[IBIS Ver]   3.2
[File name]   xc7455a-d.ibs
[File Rev]   0.1
[Date]   Wed Sep 18 11:10:01 CDT 2002
[Source]   File originated at Somerset. Created by Joshua Siegel.
[Notes]   This IBIS model is for the Apollo 483BGA ceramic package.
|   The driver and receiver models are characterized up to
|   2.5V mode on the data bus and 2.5V mode on the L3
|   interface. The convention is apollox.ibs, where x
|   is one of the configurations of data bus/L3 bus voltage
|   modes. Following is a table of the code for bus combinations:
|   IBIS model   Bus mode   L3 mode
|   xc7455a-a.ibs  2.5V   2.5V
|   xc7455a-b.ibs  2.5V   1.8V
|   xc7455a-c.ibs  2.5V   1.5V
|   xc7455a-d.ibs  1.8V   2.5V
|   xc7455a-e.ibs  1.8V   1.8V
|   xc7455a-f.ibs  1.8V   1.5V
|   NOTE: Pullup and pulldown data are non-monotonic.
|   It is safe to ignore non-monotonicity warnings.
[Disclaimer]   This information is for modeling purposes only and
|   is not guaranteed.
[Component]   Apollo
[Manufacturer]  Motorola
[Package]
|   typ   min   max
R_pkg   0.990   0.111   1.910
L_pkg   6.110nH   0.540nH   12.0nH
C_pkg   2.170pF   0.370pF   4.36pF
[Pin]   signal_name   model_name  R_pin   L_pin   C_pin
A02   PLL_CFG0   busio   1.775   1.11e-08   3.54e-12
A03   HRESET_   busio   1.555   9.71e-09   3.04e-12
A04   L3VSEL   rcvr   1.545   9.6e-09   3.9e-12
A05   TT3   busio   1.355   8.48e-09   2.8e-12
A06   A8   busio   1.436   8.97e-09   2.82e-12
A07   A6   busio   1.404   8.71e-09   3.56e-12
A09   DX_   busio   1.099   6.81e-09   2.27e-12
A10   A10   busio   1.065   6.59e-09   2.2e-12
A12   L3_DATAP7   l3io   1.065   6.56e-09   2.72e-12
A13   L3_DATA61   l3io   1.046   6.47e-09   2.17e-12
A14   L3_DATA57   l3io   1.117   6.96e-09   2.86e-12
A15   L3_DATAP6   l3io   1.113   6.9e-09   2.3e-12
A16   L3_DATA53   l3io   1.277   7.98e-09   3.25e-12
A17   L3_DATA52   l3io   1.227   7.62e-09   2.51e-12
A18   L3_DATA48   l3io   1.428   8.89e-09   3.6e-12
A19   L3_DATA47   l3io   1.447   9.04e-09   2.84e-12
A20   L3_DATA44   l3io   1.484   9.26e-09   2.99e-12
A21   L3_DATA41   l3io   1.541   9.62e-09   3.1e-12
A22   GND   POWER   0   0   0
B01   GND   POWER   0   0   0
B02   AVDD   POWER   1.462   9.13e-09   2.87e-12
B03   OVDD   POWER   0   0   0
B04   PMON_OUT_   busio   1.396   8.7e-09   2.83e-12
B05   GND   POWER   0   0   0
B06   OSHD_   busio   1.394   8.56e-09   3.06e-12
B07   TBST_   busio   1.91   1.198e-08   4.06e-12
B08   MCP_   busio   1.139   7.1e-09   2.91e-12
B09   EXT_QUAL   busio   0.962   5.94e-09   2.01e-12
B10   CHKS_   busio   0.928   5.73e-09   1.95e-12
B12   GND   POWER   0   0   0
B13   GVDD   POWER   0   0   0
B14   GND   POWER   0   0   0
B15   GVDD   POWER   0   0   0
B16   GND   POWER   0   0   0
B17   GVDD   POWER   0   0   0
B18   GND   POWER   0   0   0
B19   GVDD   POWER   0   0   0
B20   GND   POWER   0   0   0
B21   GVDD   POWER   0   0   0
B22   L3_DATA39   l3io   1.662   1.037e-08   4.18e-12
C01   TRST_   rcvr   1.339   8.16e-09   2.68e-12
C02   PLL_CFG2   busio   1.527   9.56e-09   3.68e-12
C03   GND   POWER   0   0   0
C04   BMODE1_   busio   1.314   8.17e-09   2.67e-12
C05   OVDD   POWER   0   0   0
C06   BMODE0_   busio   0.98   6.1e-09   2.27e-12
C07   OVDD   POWER   0   0   0
C08   A4   busio   1.039   6.48e-09   2.07e-12
C09   GND   POWER   0   0   0
C10   OVDD   POWER   0   0   0
C12   L3_DATA63   l3io   0.812   5.02e-09   2.11e-12
C13   L3_DATA59   l3io   0.773   4.74e-09   1.66e-12
C14   L3_DATA56   l3io   0.816   5.01e-09   1.74e-12
C15   L3_DATA54   l3io   0.99   6.11e-09   2.53e-12
C16   L3_DATA51   l3io   1.453   9.07e-09   2.85e-12
C17   L3_CLK1   l3io   1.124   7e-09   2.87e-12
C18   L3_DATA46   l3io   1.121   6.95e-09   2.31e-12
C19   L3_DATA45   l3io   1.287   8.04e-09   3.27e-12
C20   L3_DATAP4   l3io   1.344   8.4e-09   3.42e-12
C21   GND   POWER   0   0   0
C22   L3_DATA36   l3io   1.438   8.96e-09   2.91e-12
D01   TSIZ2   busio   1.173   7.25e-09   2.4e-12
D02   OVDD   POWER   0   0   0
D04   PLL_CFG3   busio   1.174   7.25e-09   2.99e-12
D06   SYSCLK   rcvr   0.911   5.66e-09   2.09e-12
D07   GND   POWER   0   0   0
D08   SRW0_   busio   0.836   5.18e-09   2.16e-12
D09   A35   busio   0.696   4.25e-09   1.51e-12
D10   A32   busio   0.712   4.39e-09   1.86e-12
D12   GVDD   POWER   0   0   0
D13   GND   POWER   0   0   0
D14   GVDD   POWER   0   0   0
D15   GND   POWER   0   0   0
D16   GVDD   POWER   0   0   0
D17   GND   POWER   0   0   0
D18   GVDD   POWER   0   0   0
D19   GND   POWER   0   0   0
D20   L3_DATA38   l3io   1.321   8.25e-09   2.6e-12
D21   GVDD   POWER   0   0   0
D22   L3_DATA33   l3io   1.476   9.19e-09   3.72e-12
E01   TT4   busio   1.148   7.12e-09   2.36e-12
E02   GND   POWER   0   0   0
E03   OVDD   POWER   0   0   0
E04   TDI   rcvr   1.072   6.64e-09   2.22e-12
E05   GND   POWER   0   0   0
E06   PMON_IN_   busio   1.021   6.42e-09   2.04e-12
E08   A2   busio   0.818   5.09e-09   1.66e-12
E09   OVDD   POWER   0   0   0
E10   A0   busio   0.601   3.62e-09   1.58e-12
E12   L3_DATA62   l3io   0.613   3.8e-09   1.27e-12
E13   L3_DATA58   l3io   0.627   3.89e-09   1.3e-12
E14   L3_ECHO_CLK3   l3io   0.661   4.1e-09   1.36e-12
E15   L3_DATA50   l3io   0.662   4.04e-09   1.45e-12
E16   L3_DATAP5   l3io   0.754   4.62e-09   1.62e-12
E17   L3_DATA43   l3io   1.273   6.1e-09   2.4e-12
E18   L3_ECHO_CLK2   l3io   0.886   5.46e-09   1.87e-12
E19   GVDD   POWER   0   0   0
E20   L3_DATA34   l3io   1.107   6.9e-09   2.83e-12
E21   GND   POWER   0   0   0
E22   L3_ADDR15   l3io   1.271   7.91e-09   2.59e-12
F01   TT0   busio   0.934   5.77e-09   1.96e-12
F02   HPR_   busio   0.813   4.99e-09   1.73e-12
F03   CKSTP_IN_   busio   0.77   4.76e-09   2e-12
F04   TT1   busio   0.594   3.61e-09   1.32e-12
F05   OVDD   POWER   0   0   0
F06   LSSD_MODE_   rcvr   0.749   4.55e-09   1.94e-12
F07   PLL_CFG1   busio   0.712   4.42e-09   1.46e-12
F08   WAIT_   busio   0.658   4.08e-09   1.35e-12
F09   SRW1_   busio   0.683   4.24e-09   1.4e-12
F10   GND   POWER   0   0   0
F12   GND   POWER   0   0   0
F13   GVDD   POWER   0   0   0
F14   GND   POWER   0   0   0
F15   GVDD   POWER   0   0   0
F16   GND   POWER   0   0   0
F17   GVDD   POWER   0   0   0
F18   L3_DATA37   l3io   0.813   5e-09   1.73e-12
F19   GND   POWER   0   0   0
F20   L3_ADDR17   l3io   0.995   6.15e-09   2.07e-12
F21   GVDD   POWER   0   0   0
F22   L3_ADDR12   l3io   1.439   8.99e-09   2.82e-12
G01   SRESET0_   busio   0.923   5.78e-09   1.85e-12
G03   OVDD   POWER   0   0   0
G04   GND   POWER   0   0   0
G05   AP4   busio   0.522   3.23e-09   1.1e-12
G06   BVSEL   rcvr   0.626   3.85e-09   1.65e-12
G07   GND   POWER   0   0   0
G08   SMI0_   busio   0.512   3.12e-09   1.37e-12
G09   OVDD   POWER   0   0   0
G10   A34   busio   1.647   1.034e-08   3.52e-12
G12   L3_DATA60   l3io   0.389   2.39e-09   8.5e-13
G13   L3_DATA55   l3io   0.365   2.24e-09   8e-13
G14   L3_DATA49   l3io   0.788   4.91e-09   1.7e-12
G15   L3_DATA42   l3io   0.603   3.62e-09   1.29e-12
G16   L3_DATA40   l3io   1.672   1.047e-08   3.47e-12
G17   GND   POWER   0   0   0
G18   L3_DATA32   l3io   1.444   9.04e-09   3e-12
G19   GVDD   POWER   0   0   0
G20   L3_ADDR13   l3io   0.911   5.62e-09   1.92e-12
G21   GND   POWER   0   0   0
G22   L3_ADDR11   l3io   1.476   9.22e-09   2.89e-12
H01   TDO   busio   0.87   5.36e-09   1.84e-12
H02   AP3   busio   0.838   5.14e-09   1.68e-12
H03   TSIZ1   busio   0.722   4.48e-09   1.47e-12
H04   L1_TSTCLK   rcvr   0.696   4.19e-09   1.41e-12
H05   GND   POWER   0   0   0
H06   IARTRY0_   busio   0.249   1.46e-09   7.2e-13
H07   OVDD   POWER   0   0   0
H08   PLL_CFG4   busio   0.583   3.63e-09   1.43e-12
H10   IARTRY1_   busio   0.318   1.89e-09   7.9e-13
H12   GVDD   POWER   0   0   0
H13   GND   POWER   0   0   0
H14   GVDD   POWER   0   0   0
H15   GND   POWER   0   0   0
H16   L3_DATA35   l3io   0.613   3.38e-09   1.17e-12
H17   GVDD   POWER   0   0   0
H18   L3_ADDR14   l3io   0.787   4.87e-09   2.04e-12
H19   GND   POWER   0   0   0
H20   L3_ADDR10   l3io   0.915   5.64e-09   1.92e-12
H21   GVDD   POWER   0   0   0
H22   L3_ADDR7   l3io   1.337   8.28e-09   3.39e-12
J01   AP2   busio   1.009   6.29e-09   2.01e-12
J02   L2_TSTCLK   busio   0.723   4.28e-09   1.53e-12
J03   GND   POWER   0   0   0
J04   A33   busio   0.44   2.49e-09   1e-12
J05   OVDD   POWER   0   0   0
J06   INT0_   busio   0.47   2.79e-09   9.7e-13
J07   TCK   rcvr   0.139   8.2e-10   3.8e-13
J09   VDD   POWER   0   0   0
J10   GND   POWER   0   0   0
J11   VDD   POWER   0   0   0
J12   GND   POWER   0   0   0
J13   VDD   POWER   0   0   0
J14   GND   POWER   0   0   0
J15   VDD   POWER   0   0   0
J16   L3_ADDR16   l3io   0.754   4.47e-09   1.63e-12
J17   GND   POWER   0   0   0
J18   L3_ADDR8   l3io   0.735   4.54e-09   1.92e-12
J19   GVDD   POWER   0   0   0
J20   L3_ADDR6   l3io   0.941   5.81e-09   1.97e-12
J21   GND   POWER   0   0   0
J22   L3_ADDR5   l3io   1.387   8.66e-09   2.72e-12
K01   BR_   busio   0.866   5.17e-09   1.8e-12
K02   HIT_   busio   0.777   4.81e-09   2.02e-12
K03   OVDD   POWER   0   0   0
K04   TMS   rcvr   0.467   2.8e-09   1.08e-12
K05   GND   POWER   0   0   0
K06   CKSTP_OUT_   busio   0.253   1.48e-09   7.3e-13
K07   QACK_   busio   0.136   8e-10   3.7e-13
K08   TT2   busio   0.341   1.67e-09   7e-13
K09   GND   POWER   0   0   0
K10   VDD   POWER   0   0   0
K11   GND   POWER   0   0   0
K12   VDD   POWER   0   0   0
K13   GND   POWER   0   0   0
K14   VDD   POWER   0   0   0
K15   GND   POWER   0   0   0
K16   L3_ADDR9   l3io   0.612   3.81e-09   1.43e-12
K17   GVDD   POWER   0   0   0
K18   L3_ADDR4   l3io   1.147   7.16e-09   2.41e-12
K19   GND   POWER   0   0   0
K20   L3_ADDR3   l3io   0.941   5.85e-09   2.42e-12
K21   GVDD   POWER   0   0   0
K22   L3_ADDR1   l3io   1.355   8.4e-09   3.43e-12
L01   TSIZ0   busio   1.271   7.88e-09   2.5e-12
L02   WT_   busio   0.821   5.1e-09   1.66e-12
L03   TBEN   busio   0.564   3.41e-09   1.26e-12
L04   SHD0_   busio   0.527   3.22e-09   1.41e-12
L05   AP0   busio   1.096   6.88e-09   2.18e-12
L06   AP1   busio   0.948   5.56e-09   1.82e-12
L07   OVDD   POWER   0   0   0
L08   SHD1_   busio   0.253   1.54e-09   5.9e-13
L09   VDD   POWER   0   0   0
L10   GND   POWER   0   0   0
L11   VDD   POWER   0   0   0
L12   GND   POWER   0   0   0
L13   VDD   POWER   0   0   0
L14   GND   POWER   0   0   0
L15   VDD   POWER   0   0   0
L16   L3_ADDR2   l3io   1.563   9.85e-09   3.21e-12
L17   GND   POWER   0   0   0
L18   L3_ADDR0   l3io   1.722   1.083e-08   4.01e-12
L19   GVDD   POWER   0   0   0
L20   L3_CNTL0   l3io   1.334   8.33e-09   2.63e-12
L21   GND   POWER   0   0   0
L22   L3_CNTL1   l3io   1.445   9.01e-09   2.92e-12
M01   A9   busio   0.916   5.65e-09   1.92e-12
M02   A7   busio   0.805   4.57e-09   1.64e-12
M03   GND   POWER   0   0   0
M04   GBL_   busio   0.608   3.73e-09   1.6e-12
M05   OVDD   POWER   0   0   0
M06   GND   POWER   0   0   0
M07   A23   busio   0.541   3.36e-09   1.27e-12
M08   A14   busio   0.344   2.11e-09   7.6e-13
M09   GND   POWER   0   0   0
M10   VDD   POWER   0   0   0
M11   GND   POWER   0   0   0
M12   VDD   POWER   0   0   0
M13   GND   POWER   0   0   0
M14   VDD   POWER   0   0   0
M15   L3_DATA31   l3io   0.91   5.58e-09   1.83e-12
M16   L3_DATA20   l3io   1.099   6.63e-09   2.21e-12
M17   GVDD   POWER   0   0   0
M18   L3_DATA21   l3io   1.199   7.49e-09   2.5e-12
M19   GND   POWER   0   0   0
M20   L3_DATA22   l3io   1.262   7.87e-09   2.49e-12
M21   GVDD   POWER   0   0   0
M22   L3_DATA23   l3io   1.261   7.87e-09   3.21e-12
N01   CLK_OUT   busio   0.968   5.61e-09   1.94e-12
N02   A12   busio   1.051   6.5e-09   2.09e-12
N03   OVDD   POWER   0   0   0
N04   A1   busio   0.82   4.72e-09   1.68e-12
N05   A3   busio   1.337   8.39e-09   3.11e-12
N06   A16   busio   0.756   4.71e-09   1.68e-12
N07   A24   busio   0.906   5.57e-09   2e-12
N08   TA_   busio   0.373   2.29e-09   8.2e-13
N09   VDD   POWER   0   0   0
N10   GND   POWER   0   0   0
N11   VDD   POWER   0   0   0
N12   GND   POWER   0   0   0
N13   VDD   POWER   0   0   0
N14   GND   POWER   0   0   0
N15   VDD   POWER   0   0   0
N16   L3_DATA18   l3io   1.714   1.076e-08   3.82e-12
N17   GND   POWER   0   0   0
N18   L3_DATA16   l3io   0.913   5.63e-09   1.92e-12
N19   GVDD   POWER   0   0   0
N20   L3_DATA17   l3io   1.342   8.38e-09   2.64e-12
N21   GND   POWER   0   0   0
N22   L3_DATA19   l3io   1.429   8.91e-09   2.89e-12
P01   A20   busio   1.076   6.67e-09   2.23e-12
P02   DTI0   busio   0.913   5.63e-09   1.92e-12
P03   GND   POWER   0   0   0
P04   A21   busio   0.924   5.52e-09   1.8e-12
P05   TS_   busio   0.72   4.28e-09   1.42e-12
P06   DTI3   busio   0.883   5.07e-09   1.68e-12
P07   OVDD   POWER   0   0   0
P08   A13   busio   0.352   2.16e-09   7.8e-13
P09   GND   POWER   0   0   0
P10   VDD   POWER   0   0   0
P11   GND   POWER   0   0   0
P12   VDD   POWER   0   0   0
P13   GND   POWER   0   0   0
P14   VDD   POWER   0   0   0
P15   GND   POWER   0   0   0
P16   L3_DATAP3   l3io   1.165   7.26e-09   2.31e-12
P17   GVDD   POWER   0   0   0
P18   L3_DATA29   l3io   0.958   5.88e-09   2e-12
P19   GND   POWER   0   0   0
P20   L3_ECHO_CLK1   l3io   1.813   1.135e-08   4.34e-12
P21   GVDD   POWER   0   0   0
P22   L3_DATAP2   l3io   1.559   9.74e-09   3.05e-12
R01   CI_   busio   1.155   7.2e-09   2.95e-12
R02   A5   busio   0.957   5.66e-09   1.95e-12
R03   BG_   busio   0.789   4.85e-09   1.69e-12
R04   OVDD   POWER   0   0   0
R05   A18   busio   1.148   7.21e-09   2.28e-12
R06   A22   busio   0.874   5.47e-09   2.09e-12
R07   D59   busio   0.414   2.44e-09   8.8e-13
R08   DP4   busio   0.377   2.2e-09   8.1e-13
R09   D60   busio   0.845   5.26e-09   1.71e-12
R10   D28   busio   0.114   5.6e-10   4.2e-13
R11   D23   busio   0.163   9.7e-10   4.2e-13
R12   D17   busio   0.111   5.4e-10   4.1e-13
R13   D50   busio   0.179   1.01e-09   5.5e-13
R14   D2   busio   0.129   7e-10   4.3e-13
R15   GVDD   POWER   0   0   0
R16   L3_DATA11   l3io   1.166   7.27e-09   2.31e-12
R17   GND   POWER   0   0   0
R18   L3_DATA24   l3io   0.955   5.9e-09   2e-12
R19   GVDD   POWER   0   0   0
R20   L3_DATA28   l3io   1.332   8.19e-09   2.6e-12
R21   GND   POWER   0   0   0
R22   L3_DATA30   l3io   1.5   9.36e-09   3.02e-12
T01   TEA_   busio   1.299   8.11e-09   2.56e-12
T02   ARTRY_   busio   0.949   5.86e-09   1.99e-12
T03   OVDD   POWER   0   0   0
T04   GND   POWER   0   0   0
T05   DTI1   busio   1.194   7.49e-09   2.77e-12
T06   DRDY_   busio   0.761   4.44e-09   1.48e-12
T07   GND   POWER   0   0   0
T08   D33   busio   0.443   2.73e-09   9.5e-13
T09   GND   POWER   0   0   0
T10   D25   busio   0.288   1.7e-09   8.2e-13
T11   D22   busio   0.287   1.7e-09   8.2e-13
T12   D14   busio   0.235   1.33e-09   6.5e-13
T13   GND   POWER   0   0   0
T14   D1   busio   0.275   1.62e-09   7.8e-13
T15   GND   POWER   0   0   0
T16   L3_DATA7   l3io   0.898   5.59e-09   1.81e-12
T17   GVDD   POWER   0   0   0
T18   L3_DATA14   l3io   1.022   6.32e-09   2.12e-12
T19   GND   POWER   0   0   0
T20   L3_DATA25   l3io   1.448   9.06e-09   3.67e-12
T21   GVDD   POWER   0   0   0
T22   L3_DATA27   l3io   1.524   9.54e-09   3.86e-12
U01   AACK_   busio   1.398   8.65e-09   2.73e-12
U02   A11   busio   1.113   6.93e-09   2.85e-12
U03   DTI2   busio   0.92   5.68e-09   1.93e-12
U04   A26   busio   0.888   5.08e-09   1.79e-12
U05   OVDD   POWER   0   0   0
U06   A17   busio   0.715   4.11e-09   1.49e-12
U07   OVDD   POWER   0   0   0
U08   DP6   busio   0.513   3.13e-09   1.37e-12
U09   D31   busio   0.354   2.08e-09   8.7e-13
U10   D29   busio   0.433   2.62e-09   1.17e-12
U11   OVDD   POWER   0   0   0
U12   D10   busio   0.43   2.65e-09   9.2e-13
U13   D13   busio   0.415   2.51e-09   1.13e-12
U14   D5   busio   0.345   2.03e-09   8.5e-13
U15   OVDD   POWER   0   0   0
U16   L3_DATA2   l3io   0.957   5.98e-09   2.13e-12
U17   GND   POWER   0   0   0
U18   L3_DATA9   l3io   1.433   8.96e-09   3.63e-12
U19   GVDD   POWER   0   0   0
U20   L3_DATA15   l3io   1.484   9.27e-09   2.91e-12
U21   GND   POWER   0   0   0
U22   L3_DATA26   l3io   1.595   9.96e-09   3.2e-12
V01   DBG_   busio   1.345   8.4e-09   3.42e-12
V02   GND   POWER   0   0   0
V03   OVDD   POWER   0   0   0
V04   A30   busio   0.988   6.02e-09   1.96e-12
V05   GND   POWER   0   0   0
V06   D56   busio   0.749   4.59e-09   1.61e-12
V07   D32   busio   0.635   3.81e-09   1.39e-12
V08   GND   POWER   0   0   0
V09   OVDD   POWER   0   0   0
V10   D27   busio   0.558   3.45e-09   1.17e-12
V11   D21   busio   0.493   2.96e-09   1.13e-12
V12   GND   POWER   0   0   0
V13   OVDD   POWER   0   0   0
V14   D4   busio   0.496   2.98e-09   1.13e-12
V15   GND   POWER   0   0   0
V16   D53   busio   0.532   3.21e-09   1.2e-12
V17   GVDD   POWER   0   0   0
V18   L3_ECHO_CLK0   l3io   1.161   7.2e-09   2.38e-12
V19   GND   POWER   0   0   0
V20   L3_DATA12   l3io   1.502   9.4e-09   3.8e-12
V21   GVDD   POWER   0   0   0
V22   L3_CLK0   l3io   1.729   1.084e-08   4.36e-12
W01   A28   busio   1.359   8.49e-09   3.45e-12
W02   A27   busio   1.209   7.51e-09   2.48e-12
W03   A29   busio   1.074   6.65e-09   2.22e-12
W04   A15   busio   1.087   6.55e-09   2.21e-12
W05   DP5   busio   1.026   6.39e-09   2.05e-12
W06   D54   busio   0.845   5.18e-09   2.18e-12
W07   GND   POWER   0   0   0
W08   D40   busio   0.597   3.63e-09   1.33e-12
W09   D63   busio   0.673   4.14e-09   1.76e-12
W10   D24   busio   0.604   3.67e-09   1.34e-12
W11   D26   busio   0.676   4.16e-09   1.77e-12
W12   D15   busio   0.662   4.07e-09   1.74e-12
W13   D11   busio   0.613   3.73e-09   1.36e-12
W14   D49   busio   0.688   4.27e-09   1.41e-12
W15   D51   busio   0.662   4.08e-09   1.74e-12
W16   D7   busio   0.795   4.94e-09   1.61e-12
W17   GND   POWER   0   0   0
W18   L3_DATA3   l3io   1.294   8.08e-09   2.55e-12
W19   GVDD   POWER   0   0   0
W20   L3_DATA8   l3io   1.454   9.1e-09   3.69e-12
W21   GND   POWER   0   0   0
W22   L3_DATA13   l3io   1.822   1.139e-08   3.54e-12
Y01   QREQ_   busio   1.632   1.02e-08   3.19e-12
Y02   OVDD   POWER   0   0   0
Y03   GND   POWER   0   0   0
Y04   A19   busio   1.175   7.33e-09   3e-12
Y05   OVDD   POWER   0   0   0
Y06   D35   busio   0.901   5.56e-09   1.9e-12
Y07   OVDD   POWER   0   0   0
Y08   D38   busio   0.807   4.99e-09   2.09e-12
Y09   GND   POWER   0   0   0
Y10   OVDD   POWER   0   0   0
Y11   D9   busio   0.738   4.52e-09   1.59e-12
Y12   D20   busio   0.79   4.89e-09   2.05e-12
Y13   GND   POWER   0   0   0
Y14   D12   busio   0.755   4.63e-09   1.62e-12
Y15   GND   POWER   0   0   0
Y16   D47   busio   0.836   5.18e-09   2.17e-12
Y17   OVDD   POWER   0   0   0
Y18   D45   busio   0.905   5.62e-09   2.34e-12
Y19   OVDD   POWER   0   0   0
Y20   GND   POWER   0   0   0
Y21   GVDD   POWER   0   0   0
Y22   L3_DATA10   l3io   1.719   1.075e-08   3.43e-12
AA01   A31   busio   1.609   1.008e-08   4.07e-12
AA02   DP0   busio   1.463   9.12e-09   2.95e-12
AA03   A25   busio   1.386   8.67e-09   3.52e-12
AA04   OVDD   POWER   0   0   0
AA05   GND   POWER   0   0   0
AA06   D37   busio   1.045   6.47e-09   2.17e-12
AA07   D39   busio   0.993   6.17e-09   2.55e-12
AA08   DP3   busio   0.87   5.36e-09   1.84e-12
AA09   D61   busio   0.88   5.42e-09   1.86e-12
AA10   D30   busio   0.877   5.4e-09   1.85e-12
AA11   D8   busio   0.936   5.82e-09   2.41e-12
AA12   D55   busio   0.865   5.33e-09   1.83e-12
AA13   D18   busio   0.88   5.42e-09   1.86e-12
AA14   D52   busio   0.971   6.05e-09   1.94e-12
AA15   OVDD   POWER   0   0   0
AA16   D42   busio   0.913   5.63e-09   1.92e-12
AA17   GND   POWER   0   0   0
AA18   D48   busio   1.358   8.47e-09   2.67e-12
AA19   L3_DATA0   l3io   1.646   1.028e-08   3.3e-12
AA20   L3_DATA4   l3io   1.675   1.047e-08   3.35e-12
AA21   L3_DATA6   l3io   1.692   1.061e-08   4.27e-12
AA22   L3_DATAP1   l3io   1.874   1.172e-08   3.64e-12
AB01   GND   POWER   0   0   0
AB02   DP2   busio   1.548   9.53e-09   3.01e-12
AB03   DP1   busio   1.411   8.67e-09   2.83e-12
AB04   D34   busio   1.312   8.16e-09   2.67e-12
AB05   DP7   busio   1.264   7.89e-09   3.22e-12
AB06   D58   busio   1.107   6.86e-09   2.28e-12
AB07   D36   busio   1.032   6.38e-09   2.14e-12
AB08   D62   busio   1.1   6.85e-09   2.82e-12
AB09   D57   busio   1.103   6.88e-09   2.19e-12
AB10   D41   busio   1.083   6.75e-09   2.15e-12
AB11   D19   busio   1.031   6.38e-09   2.14e-12
AB12   D16   busio   1.076   6.71e-09   2.14e-12
AB13   D3   busio   1.108   6.9e-09   2.2e-12
AB14   D6   busio   1.056   6.57e-09   2.71e-12
AB15   D0   busio   1.006   6.22e-09   2.09e-12
AB16   D43   busio   1.094   6.81e-09   2.8e-12
AB17   D44   busio   1.074   6.65e-09   2.22e-12
AB18   D46   busio   1.118   6.93e-09   2.3e-12
AB19   L3_DATAP0   l3io   1.756   1.098e-08   3.5e-12
AB20   L3_DATA1   l3io   1.808   1.13e-08   3.52e-12
AB21   L3_DATA5   l3io   1.903   1.19e-08   3.69e-12
AB22   GND   POWER   0   0   0
| Models and submodels in the file (3): busio (I/O), rcvr (Input), l3io (I/O)
